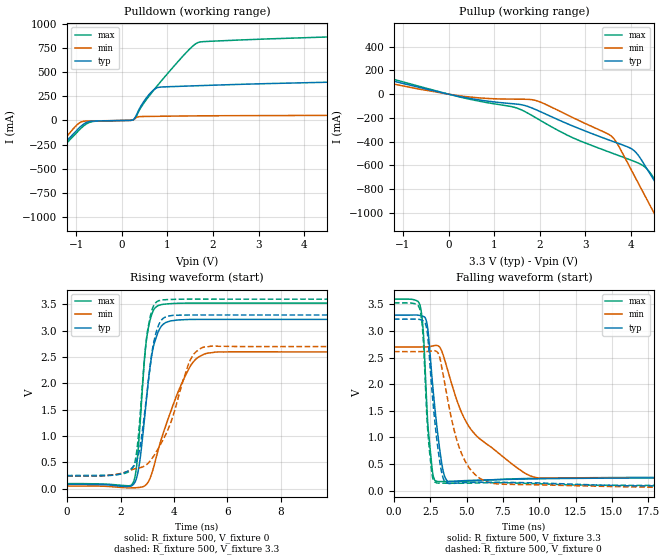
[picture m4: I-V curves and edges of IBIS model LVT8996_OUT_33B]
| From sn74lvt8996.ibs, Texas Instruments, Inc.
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[Model]   LVT8996_OUT_33B
Model_type  Output
Vref =   0
Rref =   500
Cref =   50p
Vmeas =   1.5
| variable   typ   min   max
C_comp   7.89pF   0.34pF   21.55pF
| C_pullup   7.55pF   0.34pF   21.55pF
| C_pulldown   8.23pF   1.62pF   16.10pF
[Temperature Range]   40   -40   100
| Ambient temperature   25   -40   85
[Voltage range]   3.3   2.7   3.6
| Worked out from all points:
|   slope of the pulldown table from 0 to 0.495 V, typ, clamps not added: 2.42 ohm
|   slope of the pullup table from 0 to 0.495 V, typ, clamps not added: 13.2 ohm
|   rising waveform, R_fixture 500, V_fixture 0: 20-80 % time 420ps typ, 1.05ns min, 307ps max; typ from 0.084 V to 3.22 V
|   falling waveform, R_fixture 500, V_fixture 3.3: 20-80 % time 660ps typ, 3.32ns min, 408ps max; typ from 3.3 V to 0.242 V
|   rising waveform, R_fixture 500, V_fixture 3.3: 20-80 % time 459ps typ, 1.06ns min, 339ps max; typ from 0.243 V to 3.3 V
|   falling waveform, R_fixture 500, V_fixture 0: 20-80 % time 652ps typ, 1.44ns min, 413ps max; typ from 3.22 V to 0.085 V
[Pulldown]
| LVT8996_OUT_33B
|   Voltage   I(typ)   I(min)   I(max)
-5.5V     -3.193A    -3.542A    -3.422A
-2.435V   -1.097A    -1.197A    -1.237A
-2.32V    -1.004A    -1.065A    -1.136A
-1.85V    -604mA     -534.6mA   -703.6mA
-1.46V    -334.6mA   -306.2mA   -370mA
-925mV    -72.47mA   -23.91mA   -94.75mA
-650mV    -6.987mA   -4.412mA   -12.07mA
270mV     15.72mA    12.27mA    11.67mA
515mV     217.6mA    41.36mA    199.7mA
760mV     335.2mA    42.87mA    347.5mA
1.69V     359.7mA    47.8mA     808.1mA
11V       465mA      61.55mA    962.3mA
[Pullup]
| LVT8996_OUT_33B
|   Voltage   I(typ)   I(min)   I(max)
-5.5V     511mA      451.9mA    554.3mA
-635mV    56.31mA    41.96mA    65.28mA
465mV     -35.44mA   -23.82mA   -42.68mA
1.435V    -81.32mA   -41.71mA   -109.8mA
2.04V     -151.7mA   -70.79mA   -227.2mA
2.745V    -271.3mA   -201.2mA   -370.8mA
3.6V      -397.6mA   -363.9mA   -498.4mA
4.1V      -487.4mA   -705.2mA   -570.5mA
4.35V     -628.1mA   -887.1mA   -629.8mA
4.645V    -811.4mA   -1.102A    -797.6mA
5.16V     -1.131A    -1.47A     -1.125A
11V       -4.66A     -5.595A    -4.822A
[Ramp]
| LVT8996_OUT_33B
| variable   typ   min   max
dV/dt_r   1.90/4.37E-10   1.55/1.07E-09   2.08/3.22E-10
dV/dt_f   1.88/6.86E-10   1.50/3.33E-09   2.06/4.29E-10
R_load = 500
[Rising Waveform]
| LVT8996_OUT_33B
R_fixture =   500
C_fixture =   0
L_fixture =   0
V_fixture =   0
V_fixture_min = 0
V_fixture_max = 0
|   Time   V(typ)   V(min)   V(max)
0s        84.12mV    51.14mV    97.75mV
2.47ns    78.52mV    18.02mV    116mV
2.63ns    263.7mV    22.14mV    568.5mV
2.905ns   1.376V     56.12mV    2.519V
2.99ns    1.8V       96.69mV    2.898V
3.215ns   2.662V     366.1mV    3.37V
3.52ns    3.082V     933.8mV    3.496V
4.56ns    3.214V     2.281V     3.525V
5.275ns   3.217V     2.577V     3.525V
24.99ns   3.217V     2.599V     3.525V
[Falling Waveform]
| LVT8996_OUT_33B
R_fixture =   500
C_fixture =   0
L_fixture =   0
V_fixture =   3.3
V_fixture_min = 2.7
V_fixture_max = 3.6
|   Time   V(typ)   V(min)   V(max)
0s        3.3V       2.7V       3.6V
1.805ns   3.292V     2.701V     3.475V
2.035ns   3.274V     2.702V     2.92V
2.315ns   3.071V     2.703V     1.32V
2.85ns    1.465V     2.729V     182.9mV
3.36ns    402.3mV    2.572V     171.7mV
3.705ns   171.8mV    2.259V     172.8mV
5.33ns    193mV      1.139V     181.5mV
9.36ns    220mV      280.3mV    229.2mV
24.99ns   241.8mV    240.7mV    250.4mV
[Rising Waveform]
| LVT8996_OUT_33B
R_fixture =   500
C_fixture =   0
L_fixture =   0
V_fixture =   3.3
V_fixture_min = 2.7
V_fixture_max = 3.6
|   Time   V(typ)   V(min)   V(max)
0s        243.4mV    240.9mV    251.8mV
2.465ns   412.1mV    369.8mV    409.2mV
2.64ns    591.5mV    390.3mV    858mV
3.015ns   1.931V     476.6mV    3.011V
3.21ns    2.693V     598.1mV    3.445V
3.44ns    3.127V     789.4mV    3.573V
3.91ns    3.289V     1.301V     3.595V
4.565ns   3.299V     2.397V     3.601V
5.145ns   3.3V       2.693V     3.601V
24.99ns   3.3V       2.7V       3.6V
[Falling Waveform]
| LVT8996_OUT_33B
R_fixture =   500
C_fixture =   0
L_fixture =   0
V_fixture =   0
V_fixture_min = 0
V_fixture_max = 0
|   Time   V(typ)   V(min)   V(max)
0s        3.223V     2.613V     3.529V
1.8ns     3.215V     2.614V     3.397V
2.01ns    3.193V     2.614V     2.876V
2.425ns   2.563V     2.618V     800.6mV
2.655ns   1.756V     2.629V     254.4mV
2.89ns    1.108V     2.623V     150.3mV
3.52ns    161.7mV    1.981V     139.7mV
4.665ns   148.2mV    687.8mV    139mV
6.285ns   157.6mV    176.6mV    147.4mV
24.99ns   84.68mV    52.17mV    98.16mV
